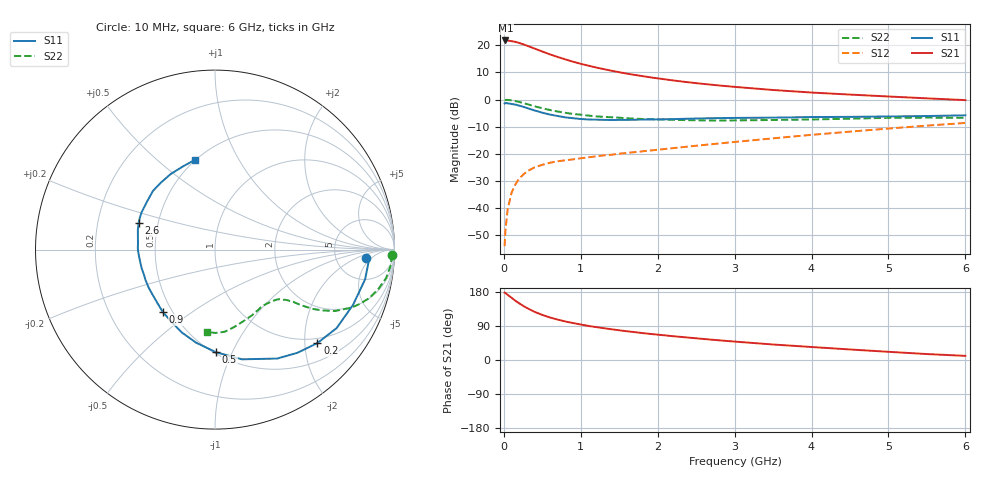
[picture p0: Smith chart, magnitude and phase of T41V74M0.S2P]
! Infineon Technologies  Discrete & RF Semiconductors
! BFR182T
! Si NPN RF Bipolar Junction Transistor in SC75
! VCE = 1.75 V  IC = 4 mA
! Common Emitter S-Parameters:  October  1999
# GHz  S  MA  R  50
!  f  S11  S21  S12  S22
! GHz  MAG  ANG  MAG  ANG  MAG  ANG  MAG  ANG
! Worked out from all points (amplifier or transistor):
!   36 points, 10 MHz to 6 GHz, reference 50 ohm
!   highest |S21| = 21.7 dB at 20 MHz (marker M1)
!   |S21| within 3 dB of that: start of sweep to 401.7 MHz
!   unconditionally stable (mu >= 1): 1.512 GHz to 4.124 GHz
!   at 250 MHz: K = 0.24, MSG = 24.0 dB, |S12| = -27.7 dB
!   at 1.4 GHz: K = 0.98, MSG = 15.5 dB, |S12| = -20.3 dB
!   at 6 GHz: K = 0.85, MSG = 4.2 dB, |S12| = -8.6 dB
!   S11 on the Smith chart (normalised r, x): 10 MHz: 11, -4; 200 MHz: 0.88, -2.29; 500 MHz: 0.51, -0.87; 900 MHz: 0.44, -0.39; 2.6 GHz: 0.39, +0.14; 6 GHz: 0.50, +0.67
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0.01  0.845 -3.3  12.18 177.7  0.002 80.8  0.9853 -1.7
0.02  0.861 -3.3  12.22 177.0  0.0038 92.7  0.9833 -1.9
0.05  0.8526 -11.2  12.17 171.8  0.0096 82.9  0.9845 -4.8
0.1  0.8284 -21.8  11.86 164.3  0.0192 79.4  0.9668 -9.4
0.15  0.8066 -32.8  11.5 156.4  0.0274 73.6  0.936 -13.6
0.2  0.7726 -42.4  11 149.5  0.0353 69.5  0.9025 -17.3
0.25  0.7358 -51.4  10.4 143.1  0.0412 64.9  0.863 -20.5
0.3  0.6989 -60.3  9.801 137.2  0.0475 61.6  0.825 -23.1
0.4  0.6294 -76.2  8.669 127.0  0.0565 55.9  0.7509 -27.1
0.5  0.5721 -89.4  7.65 119.0  0.0628 52.9  0.6908 -29.4
0.6  0.5291 -101.5  6.771 112.2  0.0687 50.8  0.6414 -31.1
0.7  0.4971 -111.9  6.066 106.6  0.073 49.7  0.6007 -32.1
0.8  0.4692 -121.4  5.479 101.6  0.0763 48.9  0.569 -32.9
0.9  0.4532 -130.0  4.961 97.5  0.0792 49.0  0.5424 -33.4
1.1  0.429 -144.4  4.196 89.9  0.0866 49.1  0.5063 -34.5
1.6  0.4223 -170.7  2.995 75.8  0.104 52.2  0.4522 -37.7
2.2  0.4358 170.3  2.246 62.8  0.1274 56.3  0.4237 -43.8
2.6  0.4506 161.0  1.934 55.4  0.1457 58.1  0.4132 -48.7
3.5  0.4642 144.3  1.497 40.9  0.193 59.7  0.4204 -61.0
4.5  0.4797 129.0  1.233 27.8  0.2565 58.0  0.4438 -75.8
5.5  0.4966 111.2  1.051 15.7  0.331 53.6  0.4644 -89.5
6  0.5124 102.6  0.975 10.9  0.3705 50.3  0.4616 -95.5
